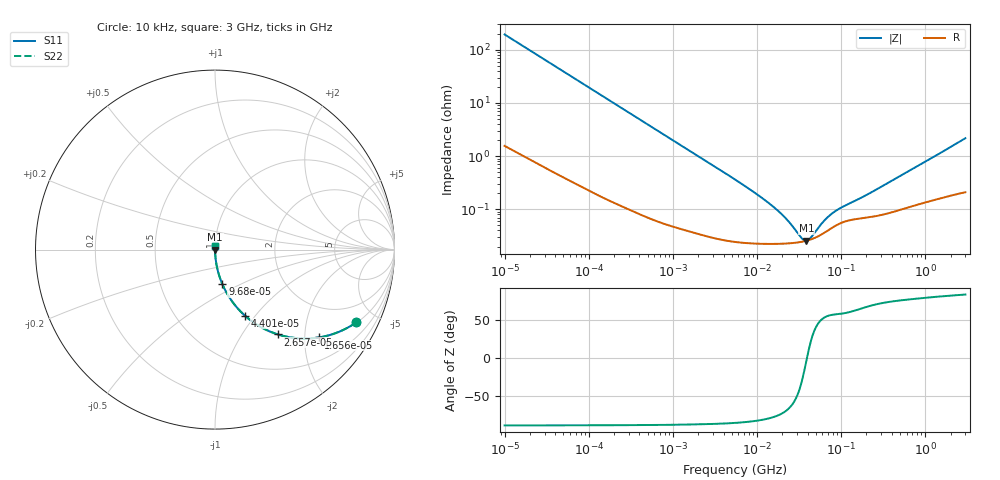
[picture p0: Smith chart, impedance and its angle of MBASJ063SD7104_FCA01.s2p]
! MBASJ063SD7104_FCA01  S-PARAMETER MODEL  ( Standard Model )
! Model Generated by TAIYO YUDEN Corporation (http://www.ty-top.com)
! Version 1.0
! TAIYO YUDEN Control No. 220601
! Copyright(c) 2020 TAIYO YUDEN CO.,LTD. All Rights Reserved.
! Product Description (link to TY-COMPAS)
! https://ds.yuden.co.jp/TYCOMPAS/or/detail?pn=MBASJ063SD7104KFCA01&u=M
! Products Name : Multilayer Ceramic Capacitors
! Characteristics :
!  Capacitance : 0.1 [uF] , Rated Voltage : 6.3 [V] , TCC : X7T
!  Case Size : 0.6 x 0.3 / 0.024 x 0.012 [mm/inch] , Thickness : 0.3 / 0.012 [mm/inch]
!  (Conditions: Temperature = 25 [degC] , DC Bias Voltage = 0 [V])
! External Node Assignments :
!  1  o---| |---o  2
! GND o---------o GND
! Frequency Range : 10kHz  -  3GHz  [ 401 STEP ]
# MHZ S RI R 50
! Freq[MHz].  S11 Real  S11 Imag  S21 Real  S21 Imag  S12 Real  S12 Imag  S22 Real  S22 Imag
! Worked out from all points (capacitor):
!   401 points, 10 kHz to 3 GHz, reference 50 ohm
!   read as one part in series: C = 82.1 nF near 10.65 kHz
!   lowest |Z| = 25.7 mohm at 38.68 MHz (marker M1)
!   series resonance near 39.23 MHz, so ESL is about 200 pH
!   S11 on the Smith chart (normalised r, x): 10 kHz: 1.03, -3.87; 16.56 kHz: 1.02, -2.34; 26.57 kHz: 1.01, -1.46; 44.01 kHz: 1.01, -0.89; 96.8 kHz: 1.00, -0.41; 3 GHz: 1.00, +0.04
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0.01  0.7877 -0.405  0.2123 0.405  0.2123 0.405  0.7877 -0.405
0.012083  0.7186 -0.4456  0.2814 0.4456  0.2814 0.4456  0.7186 -0.4456
0.016561  0.5782 -0.4895  0.4218 0.4895  0.4218 0.4895  0.5782 -0.4895
0.026575  0.3505 -0.4725  0.6495 0.4725  0.6495 0.4725  0.3505 -0.4725
0.044011  0.1669 -0.3679  0.8331 0.3679  0.8331 0.3679  0.1669 -0.3679
0.058452  0.1032 -0.299  0.8968 0.299  0.8968 0.299  0.1032 -0.299
0.082683  0.0554 -0.2233  0.9446 0.2233  0.9446 0.2233  0.0554 -0.2233
0.096801  0.0415 -0.1938  0.9585 0.1938  0.9585 0.1938  0.0415 -0.1938
0.226771  0.0087 -0.0862  0.9913 0.0862  0.9913 0.0862  0.0087 -0.0862
0.683653  0.00142 -0.029  0.9986 0.029  0.9986 0.029  0.00142 -0.029
5.477226  0.000257 -0.00363  0.9997 0.00363  0.9997 0.00363  0.000257 -0.00363
10.61963  0.000228 -0.00177  0.9998 0.00177  0.9998 0.00177  0.000228 -0.00177
16.51234  0.000225 -0.00102  0.9998 0.00102  0.9998 0.00102  0.000225 -0.00102
23.35767  0.000229 -0.000565  0.9998 0.000565  0.9998 0.000565  0.000229 -0.000565
34.09912  0.000245 -0.000147  0.9998 0.000147  0.9998 0.000147  0.000245 -0.000147
38.68249  0.000256 -1.45e-05  0.9997 1.45e-05  0.9997 1.45e-05  0.000256 -1.45e-05
41.20027  0.000264 5.14e-05  0.9997 -5.14e-05  0.9997 -5.14e-05  0.000264 5.14e-05
45.28751  0.000277 0.00015  0.9997 -0.00015  0.9997 -0.00015  0.000277 0.00015
62.07353  0.000356 0.000479  0.9996 -0.000479  0.9996 -0.000479  0.000356 0.000479
82.4407  0.000474 0.000755  0.9995 -0.000755  0.9995 -0.000755  0.000474 0.000755
374.4521  0.000862 0.00313  0.9991 -0.00313  0.9991 -0.00313  0.000862 0.00313
3000  0.00256 0.0215  0.9974 -0.0215  0.9974 -0.0215  0.00256 0.0215
